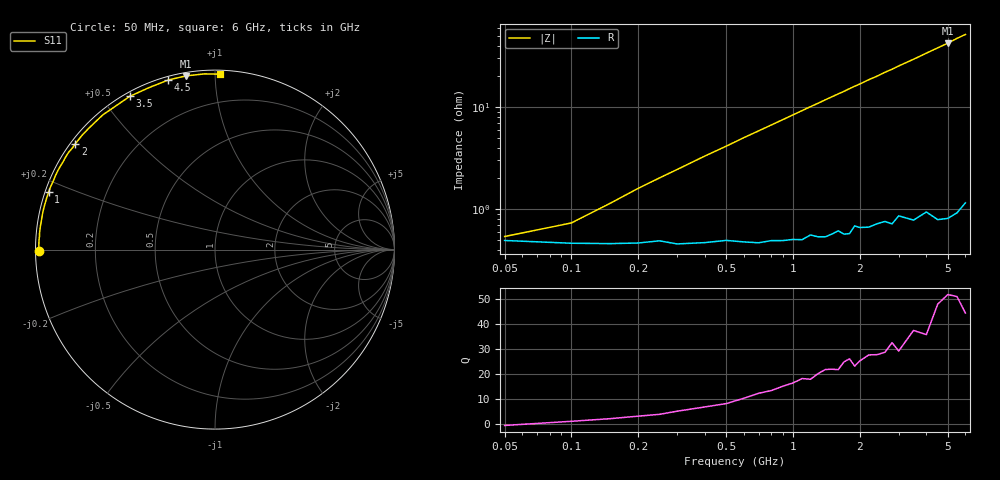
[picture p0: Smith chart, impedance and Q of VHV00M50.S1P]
! Infineon Technologies  Discrete & RF Semiconductors
! BB 814
! Si Tuning Diode in SOT23
! VR =
! S-Parameters:  July  1999
# GHz  S  MA  R  50
!  f  S11
! GHz  MAG  ANG
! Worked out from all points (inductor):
!   34 points, 50 MHz to 6 GHz, reference 50 ohm
!   read as one part to ground: L = 1.25 nH near 200 MHz
!   highest Q = 51.2 at 5 GHz (marker M1), where L = 1.34 nH
!   S11 on the Smith chart (normalised r, x): 50 MHz: 0.01, -0.00; 1 GHz: 0.01, +0.17; 2 GHz: 0.01, +0.34; 3.5 GHz: 0.02, +0.59; 4.5 GHz: 0.02, +0.76; 6 GHz: 0.02, +1.03
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0.05  0.9805 -179.5
0.1  0.9816 178.7
0.2  0.9815 176.5
0.3  0.9819 174.5
0.4  0.9814 172.5
0.7  0.9817 166.7
0.8  0.9808 164.8
1  0.9805 161.0
1.1  0.9807 159.1
1.2  0.9788 157.2
1.3  0.9798 155.4
1.4  0.9799 153.5
1.6  0.9774 149.9
1.7  0.9791 148.2
1.8  0.9791 146.3
1.9  0.9754 144.5
2  0.9765 142.9
2.2  0.9768 139.3
2.4  0.9755 136.2
2.6  0.9749 132.7
2.8  0.9768 129.7
3  0.973 126.4
3.5  0.977 119.1
4  0.9745 112.0
4.5  0.9802 105.5
5  0.9812 99.6
5.5  0.9807 93.4
6  0.9778 88.4
